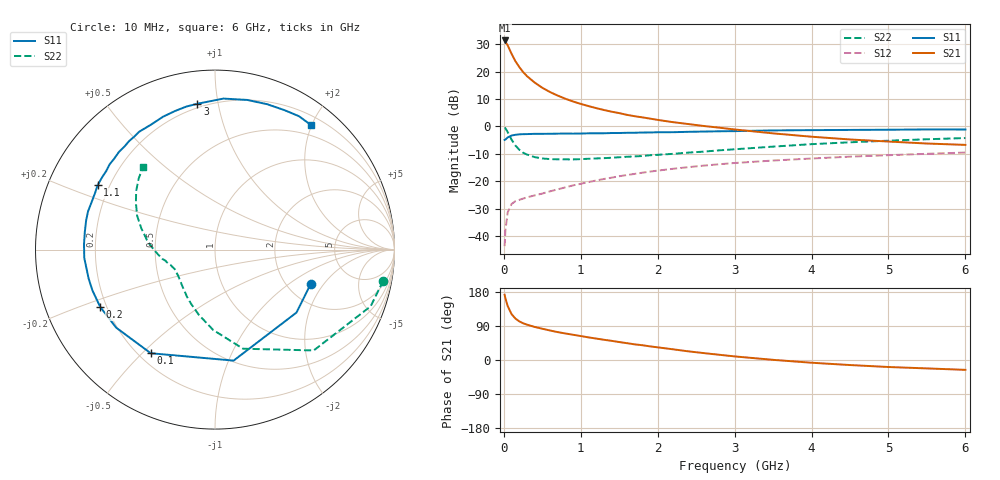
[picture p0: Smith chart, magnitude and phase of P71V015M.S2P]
! SIEMENS Small Signal Semiconductors
! BFP196
! Si NPN RF Bipolar Junction Transistor in SOT143
! VCE = 1 V  IC = 15 mA
! Common Emitter S-Parameters:  May  1996
# GHz  S  MA  R  50
!  f  S11  S21  S12  S22
! GHz  MAG  ANG  MAG  ANG  MAG  ANG  MAG  ANG
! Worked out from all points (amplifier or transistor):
!   36 points, 10 MHz to 6 GHz, reference 50 ohm
!   highest |S21| = 31.4 dB at 10 MHz (marker M1)
!   |S21| within 3 dB of that: start of sweep to 69.81 MHz
!   unconditionally stable (mu >= 1): 729.4 MHz to 5.275 GHz; 5.728 GHz to end of sweep
!   at 250 MHz: K = 0.53, MSG = 23.1 dB, |S12| = -26.4 dB
!   at 1.4 GHz: K = 1.14, MAG = 9.8 dB, |S12| = -18.7 dB
!   at 6 GHz: K = 1.01, MAG = 0.9 dB, |S12| = -9.6 dB
!   S11 on the Smith chart (normalised r, x): 10 MHz: 2.68, -1.50; 100 MHz: 0.25, -0.53; 200 MHz: 0.18, -0.23; 1.1 GHz: 0.15, +0.25; 3 GHz: 0.18, +0.87; 6 GHz: 0.33, +1.99
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0.01  0.5668 -19.6  36.98 172.1  0.0065 81.8  0.9533 -10.5
0.02  0.5737 -37.7  35.26 162.9  0.0125 75.8  0.923 -20.0
0.05  0.6271 -80.5  30.09 142.4  0.0269 57.6  0.7864 -45.6
0.1  0.6794 -121.8  21.18 121.1  0.0382 42.9  0.5739 -74.2
0.15  0.7016 -141.7  15.48 109.4  0.0431 36.2  0.4478 -91.3
0.2  0.7148 -153.4  12.14 102.1  0.0455 34.5  0.3752 -103.8
0.25  0.7199 -161.6  9.828 97.0  0.048 34.6  0.3309 -113.6
0.3  0.7224 -167.2  8.274 93.3  0.0505 35.5  0.3063 -120.5
0.4  0.7299 -176.4  6.307 87.3  0.0549 37.4  0.2744 -131.2
0.5  0.7304 177.7  5.06 82.5  0.0593 40.4  0.2594 -138.7
0.6  0.7319 172.3  4.232 77.9  0.0651 42.6  0.2525 -143.9
0.7  0.7361 167.3  3.645 73.6  0.0708 43.8  0.2501 -148.0
0.9  0.7367 158.9  2.842 66.6  0.0837 46.2  0.2493 -153.8
1.1  0.7458 151.3  2.345 59.7  0.0961 47.1  0.2561 -157.8
1.3  0.7477 144.1  1.991 53.4  0.1094 47.0  0.2627 -161.3
1.6  0.7631 134.6  1.623 44.4  0.1292 45.6  0.2784 -165.6
2.2  0.7821 117.2  1.192 28.2  0.1681 40.5  0.3151 -174.3
3  0.8184 96.9  0.877 9.5  0.2142 31.3  0.3814 172.3
3.5  0.8427 86.8  0.745 0.4  0.2378 25.1  0.4267 164.0
4.5  0.8606 70.3  0.576 -13.3  0.2797 13.8  0.5119 149.4
5.5  0.8783 57.8  0.486 -22.2  0.3155 3.1  0.5814 137.0
6  0.876 52.4  0.459 -26.0  0.3325 -2.8  0.6114 130.9
